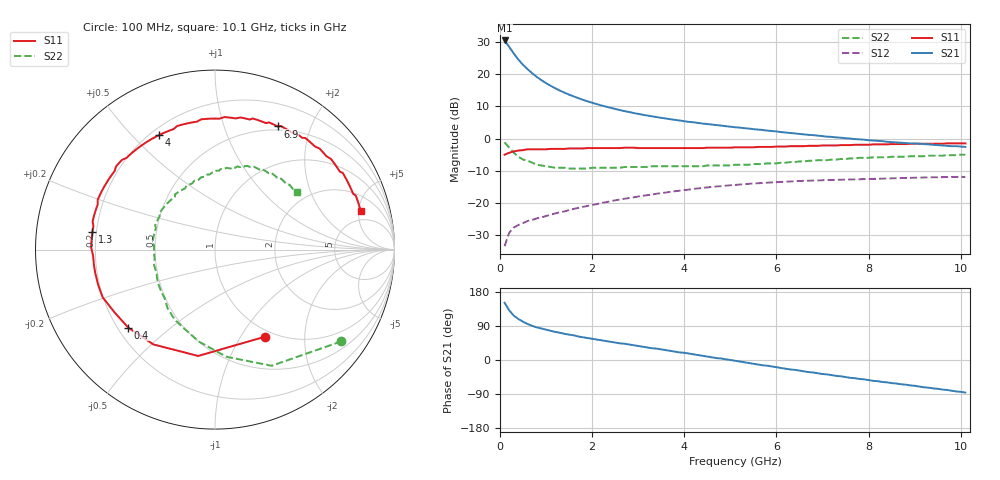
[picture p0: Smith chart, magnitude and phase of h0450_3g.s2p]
!HBFP-0450
!S and NOISE PARAMETERS at Vce=3V  Ic=35mA.  LAST UPDATED  09-04-98
# GHZ S MA R  50
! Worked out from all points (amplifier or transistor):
!   101 points, 100 MHz to 10.1 GHz, reference 50 ohm
!   highest |S21| = 30.6 dB at 100 MHz (marker M1)
!   |S21| within 3 dB of that: start of sweep to 247.5 MHz
!   unconditionally stable (mu >= 1): 2.308 GHz to end of sweep
!   at 1.7 GHz: K = 0.92, MSG = 17.1 dB, |S12| = -21.6 dB
!   at 5.1 GHz: K = 1.09, MAG = 7.2 dB, |S12| = -14.5 dB
!   at 10.1 GHz: K = 1.07, MAG = 3.1 dB, |S12| = -12.0 dB
!   lowest NFmin = 1.49 dB at 1.8 GHz
!   S11 on the Smith chart (normalised r, x): 100 MHz: 0.91, -1.29; 400 MHz: 0.24, -0.36; 1.3 GHz: 0.18, +0.07; 4 GHz: 0.23, +0.60; 6.9 GHz: 0.46, +1.54; 10.1 GHz: 3.55, +5.25
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0.1  0.56 -60.0  33.79 151.0  0.021 66.0  0.87 -36.0
0.2  0.6 -99.0  26.81 131.0  0.034 51.0  0.72 -64.0
0.3  0.63 -123.0  21.09 117.0  0.041 44.0  0.6 -84.0
0.4  0.65 -138.0  16.99 108.0  0.045 40.0  0.52 -100.0
0.5  0.66 -148.0  14.08 101.0  0.048 38.0  0.47 -112.0
0.6  0.68 -157.0  12.03 95.0  0.052 36.0  0.45 -120.0
0.7  0.68 -163.0  10.39 90.0  0.054 36.0  0.42 -129.0
0.8  0.68 -169.0  9.12 86.0  0.057 36.0  0.39 -136.0
1  0.68 -177.0  7.3 80.0  0.062 37.0  0.37 -148.0
1.2  0.69 175.0  6.07 74.0  0.068 37.0  0.35 -158.0
1.3  0.69 172.0  5.59 72.0  0.071 37.0  0.35 -163.0
1.5  0.7 167.0  4.83 67.0  0.077 37.0  0.34 -171.0
1.8  0.7 159.0  4.01 60.0  0.086 37.0  0.34 179.0
2.2  0.71 150.0  3.28 52.0  0.099 34.0  0.35 169.0
2.6  0.71 142.0  2.78 44.0  0.112 32.0  0.35 160.0
3.5  0.71 125.0  2.1 28.0  0.141 23.0  0.37 143.0
4  0.71 116.0  1.86 19.0  0.157 17.0  0.37 135.0
5.1  0.73 96.0  1.5 -2.0  0.189 3.0  0.39 114.0
6.8  0.77 65.0  1.13 -33.0  0.221 -22.0  0.45 84.0
6.9  0.77 63.0  1.11 -35.0  0.222 -23.0  0.46 82.0
8.5  0.82 38.0  0.88 -61.0  0.24 -45.0  0.52 60.0
10.1  0.84 15.0  0.74 -86.0  0.252 -67.0  0.56 35.0
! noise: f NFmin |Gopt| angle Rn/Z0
1.8  1.49  0.56  -155  0.07
2  1.53  0.56  -153  0.08
2.5  1.67  0.58  -142  0.13
3.5  1.94  0.62  -125  0.26
4  2.1  0.64  -114  0.39
5  2.38  0.67  -95  0.72
5.5  2.53  0.7  -85  1
7  2.96  0.75  -58  2.06
8  3.24  0.79  -42  3.02
10  3.81  0.8  -13  4.85
